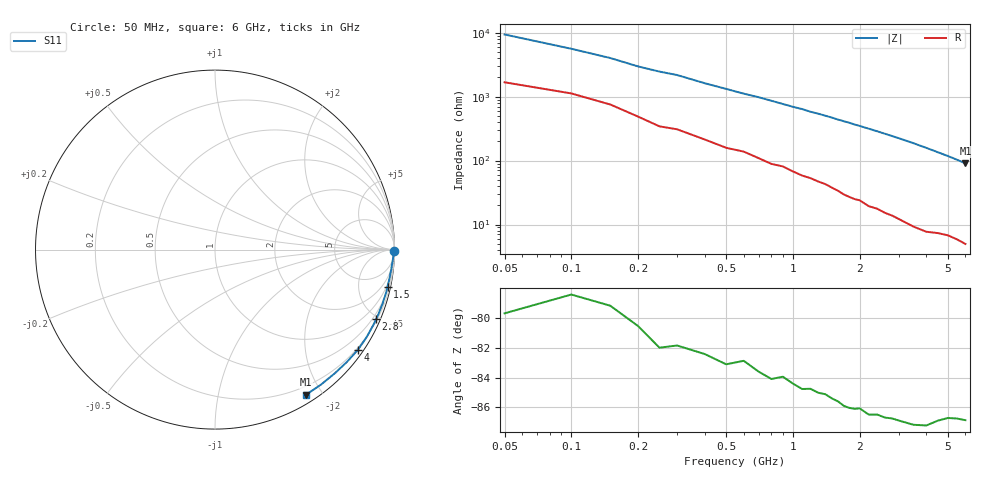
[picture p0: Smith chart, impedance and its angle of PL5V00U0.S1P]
! Infineon Technologies  Discrete & RF Semiconductors
! BAR 64-04W /-05W /-06W
! Si PIN Diode in SOT323
! VR = 5 V
! S-Parameters:  October  2008
# GHz  S  MA  R  50
!  f  S11
! GHz  MAG  ANG
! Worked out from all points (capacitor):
!   34 points, 50 MHz to 6 GHz, reference 50 ohm
!   read as one part to ground: C = 289 fF near 50 MHz
!   lowest |Z| = 90.5 ohm at 6 GHz (marker M1)
!   S11 on the Smith chart (normalised r, x): 50 MHz: open; 1.5 GHz: 0.75, -9.38; 2.8 GHz: 0.28, -4.84; 4 GHz: 0.15, -3.16; 6 GHz: 0.10, -1.81
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0.05  0.9981 -0.6
0.15  0.9953 -1.4
0.2  0.9945 -1.9
0.25  0.9944 -2.3
0.3  0.9935 -2.6
0.4  0.9919 -3.5
0.6  0.989 -5.1
0.7  0.9887 -5.8
0.8  0.9882 -6.6
1  0.9861 -8.2
1.1  0.9859 -8.9
1.2  0.9845 -9.8
1.3  0.9842 -10.5
1.5  0.9833 -12.1
1.6  0.9829 -13.0
1.8  0.9827 -14.6
1.9  0.9819 -15.5
2.2  0.9812 -18.0
2.4  0.9795 -19.7
2.6  0.979 -21.5
2.8  0.9777 -23.3
3  0.9771 -25.1
3.5  0.9756 -29.9
4  0.9723 -35.1
4.5  0.9653 -40.5
5  0.9595 -45.9
5.5  0.9563 -51.7
6  0.9545 -57.8
